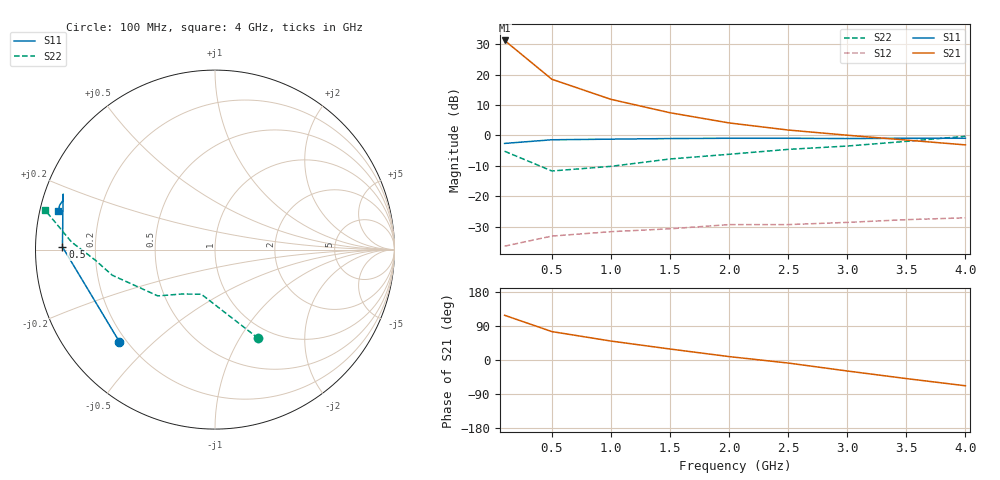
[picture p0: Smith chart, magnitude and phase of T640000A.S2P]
!AT-64000
!S-PARAMETERS at Vce=12V  Ic=110mA.  LAST UPDATED 07-13-94
# ghz s ma r 50
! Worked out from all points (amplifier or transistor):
!   9 points, 100 MHz to 4 GHz, reference 50 ohm
!   highest |S21| = 31.3 dB at 100 MHz (marker M1)
!   |S21| within 3 dB of that: start of sweep to 193.8 MHz
!   unconditionally stable (mu >= 1): nowhere
!   at 500 MHz: K = 0.59, MSG = 25.8 dB, |S12| = -33.2 dB
!   at 2 GHz: K = 0.94, MSG = 16.8 dB, |S12| = -29.4 dB
!   at 4 GHz: K = -0.36, MSG = 12.0 dB, |S12| = -27.1 dB
!   S11 on the Smith chart (normalised r, x): 100 MHz: 0.17, -0.39; 500 MHz: 0.08, +0.01; 4 GHz: 0.05, +0.12
0.1  0.74 -136.0  36.8 118.0  0.015 39.0  0.55 -64.0
0.5  0.85 179.0  8.44 75.0  0.022 24.0  0.26 -107.0
1  0.87 167.0  3.94 50.0  0.026 23.0  0.31 -127.0
1.5  0.89 162.0  2.37 29.0  0.029 24.0  0.41 -141.0
2  0.9 160.0  1.61 9.0  0.034 19.0  0.49 -156.0
2.5  0.9 160.0  1.23 -8.0  0.034 14.0  0.59 -166.0
3  0.89 162.0  1.01 -29.0  0.037 1.0  0.67 -175.0
3.5  0.9 164.0  0.84 -49.0  0.041 -6.0  0.8 177.0
4  0.9 166.0  0.7 -68.0  0.044 -9.0  0.97 167.0
